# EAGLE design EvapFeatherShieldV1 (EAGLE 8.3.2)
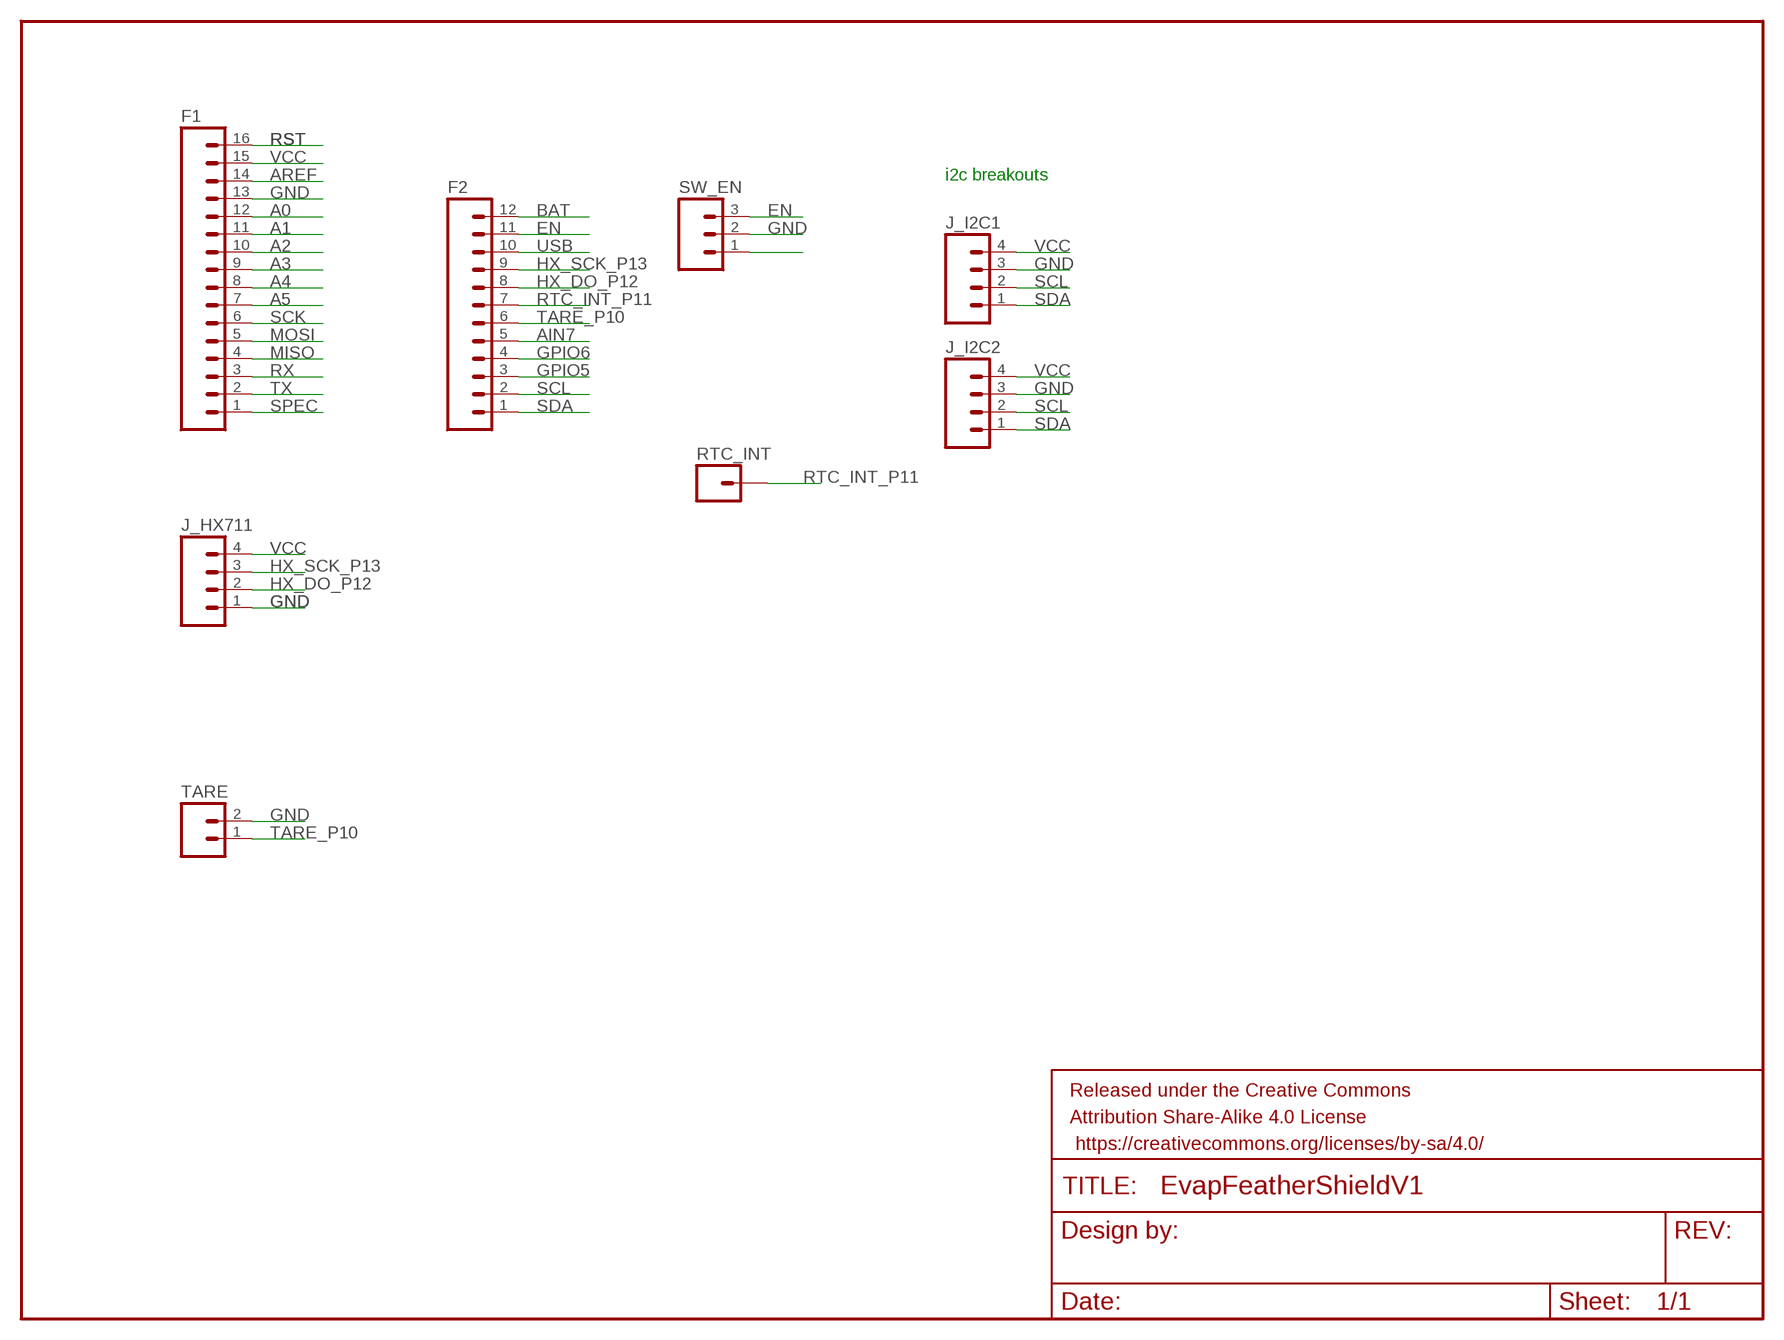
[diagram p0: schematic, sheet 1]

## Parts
F1  M16PTH  [1X16]
F2  M12PTH  [1X12]
FRAME1  FRAME-LETTER  [CREATIVE_COMMONS]
J_HX711  M04PTH  [1X04]
J_I2C1  M04PTH  [1X04]
J_I2C2  M04PTH  [1X04]
RTC_INT  M01PTH  [1X01]
SW_EN  M03PTH  [1X03]
TARE  M02PTH  [1X02]

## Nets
A0: F1.12
A1: F1.11
A2: F1.10
A3: F1.9
A4: F1.8
A5: F1.7
AIN7: F2.5
AREF: F1.14
BAT: F2.12
EN: F2.11 SW_EN.3
GND: F1.13 J_HX711.1 J_I2C1.3 J_I2C2.3 SW_EN.2 TARE.2
GPIO5: F2.3
GPIO6: F2.4
HX_DO_P12: F2.8 J_HX711.2
HX_SCK_P13: F2.9 J_HX711.3
MISO: F1.4
MOSI: F1.5
N$3: SW_EN.1
RST: F1.16
RTC_INT_P11: F2.7 RTC_INT.1
RX: F1.3
SCK: F1.6
SCL: F2.2 J_I2C1.2 J_I2C2.2
SDA: F2.1 J_I2C1.1 J_I2C2.1
SPEC: F1.1
TARE_P10: F2.6 TARE.1
TX: F1.2
USB: F2.10
VCC: F1.15 J_HX711.4 J_I2C1.4 J_I2C2.4

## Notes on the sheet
- i2c breakouts

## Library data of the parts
F1 = SparkFun-Connectors:M16: 1x16 .1" header
F2 = SparkFun-Connectors:M12: Header 12 Standard 12-pin 0.1" header. Use with straight break away headers (SKU : PRT-00116), right angle break away headers (PRT-00553), swiss pins (PRT-00743), machine pins (PRT-00117), and female headers (PRT-00115).
FRAME1 = SparkFun-Aesthetics:FRAME-LETTER: Schematic Frame
J_HX711 J_I2C1 J_I2C2 = SparkFun-Connectors:M04: Header 4 Standard 4-pin 0.1" header. Use with straight break away headers (SKU : PRT-00116), right angle break away headers (PRT-00553), swiss pins (PRT-00743), machine pins (PRT-00117), and female headers (PRT-00115). Molex polarized connector foot print use with SKU : PRT-08231 with associated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; PROD_ID: CONN-09696
RTC_INT = SparkFun-Connectors:M01: Header 1
SW_EN = SparkFun-Connectors:M03: Header 3 Standard 3-pin 0.1" header. Use with straight break away headers (SKU : PRT-00116), right angle break away headers (PRT-00553), swiss pins (PRT-00743), machine pins (PRT-00117), and female headers (PRT-00115). Molex polarized connector foot print use with SKU : PRT-08232 with associated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
TARE = SparkFun-Connectors:M02: Standard 2-pin 0.1" header. Use with

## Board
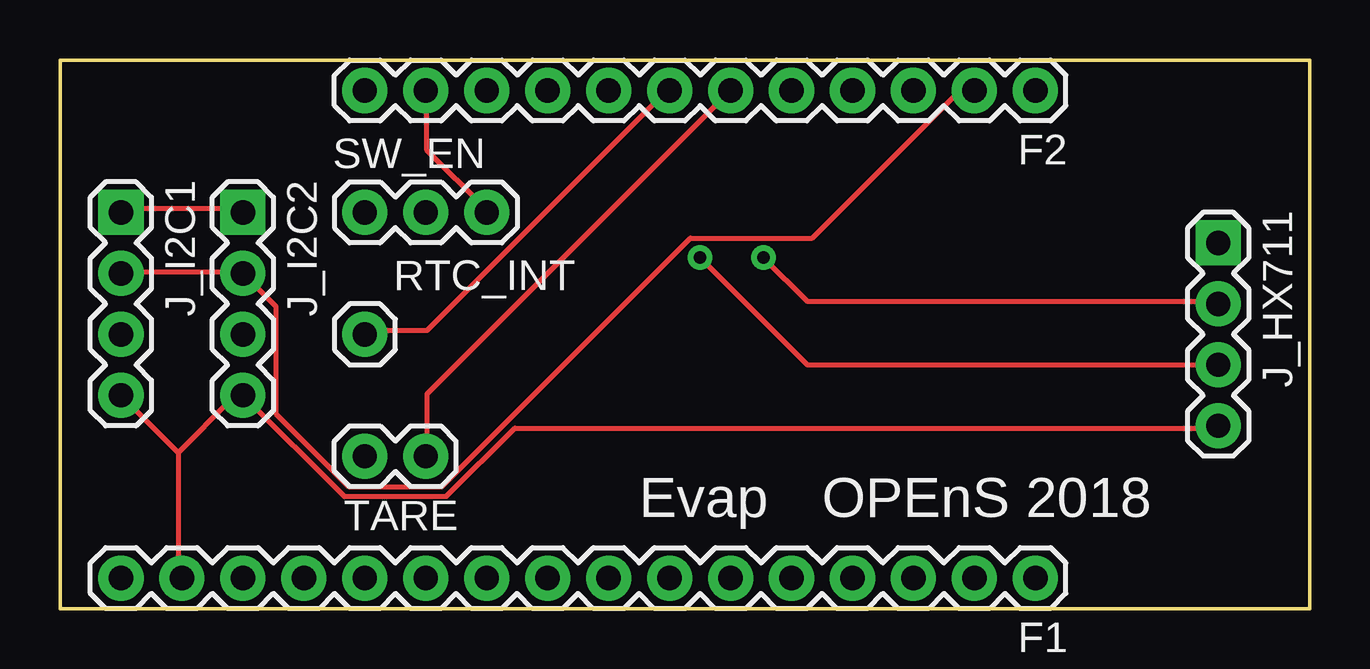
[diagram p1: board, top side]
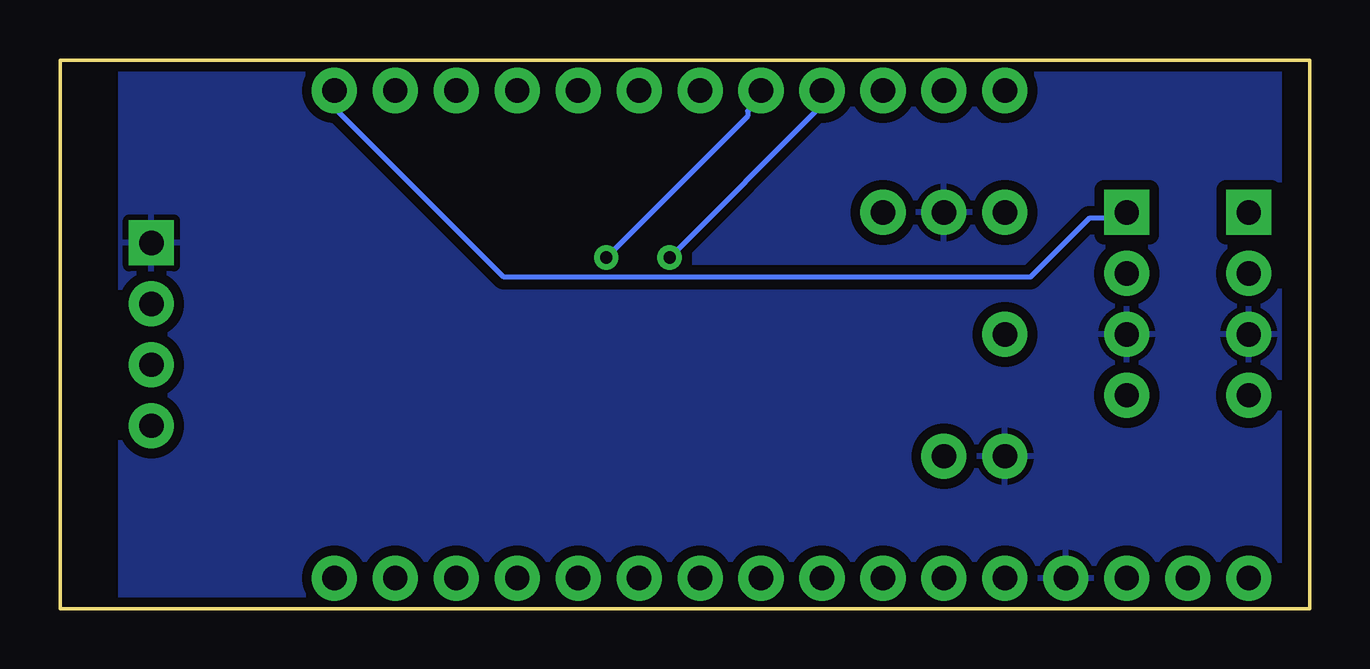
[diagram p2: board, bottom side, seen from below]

Size 52.07 x 22.86 mm. Coordinates in mm from the lower left corner, seen from the top.
Outline: 0,0 0,22.86 52.07,22.86 52.07,0 0,0
Copper layers (1*16): Top 0.035mm / dielectric 1.5mm / Bottom 0.035mm
Design rules "SparkFun": minimum track width 8mil, minimum drill 20mil, track to track 8mil, track to pad 8mil, pad to pad 8mil, via to via 8mil, smd to smd 8mil, copper to edge 8mil, drill to drill 8mil, minimum pad ring 12mil, minimum via ring 10mil, stop-mask expansion 4mil, vias tented up to drill 20mil, thermal gap 10mil

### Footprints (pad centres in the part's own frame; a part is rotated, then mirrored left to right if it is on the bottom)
1X16 = drill 1.016 pad 1.88: 1 0,0; 2 2.54,0; 3 5.08,0; 4 7.62,0; 5 10.16,0; 6 12.7,0; 7 15.24,0; 8 17.78,0; 9 20.32,0; 10 22.86,0; 11 25.4,0; 12 27.94,0; 13 30.48,0; 14 33.02,0; 15 35.56,0; 16 38.1,0
1X12 = drill 1.016 pad 1.88: 1 0,0; 2 2.54,0; 3 5.08,0; 4 7.62,0; 5 10.16,0; 6 12.7,0; 7 15.24,0; 8 17.78,0; 9 20.32,0; 10 22.86,0; 11 25.4,0; 12 27.94,0
1X04 = drill 1.016 pad 1.88 square: 1 0,0 | drill 1.016 pad 1.88: 2 2.54,0; 3 5.08,0; 4 7.62,0
1X01 = drill 1.016 pad 1.88: 1 0,0
1X03 = drill 1.016 pad 1.88: 1 0,0; 2 2.54,0; 3 5.08,0
1X02 = drill 1.016 pad 1.88: 1 0,0; 2 2.54,0

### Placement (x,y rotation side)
F1  40.64,1.27 180 top
F2  40.64,21.59 180 top
FRAME1  not placed on the board
J_HX711  48.26,15.24 270 top
J_I2C1  2.54,16.51 270 top
J_I2C2  7.62,16.51 270 top
RTC_INT  12.7,11.43 0 top
SW_EN  12.7,16.51 0 top
TARE  15.24,6.35 180 top

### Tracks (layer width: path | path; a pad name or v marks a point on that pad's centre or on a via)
EN
  Top 0.203: F2.11 15.29,21.54 15.29,19.1 17.73,16.66 SW_EN.3
GND
  pour Bottom (isolate 0.406): 1.27,0 1.27,22.86 49.53,22.86 49.53,0
HX_DO_P12  (via drill 0.51)
  Top 0.203: v29.31,14.63 31.14,12.8 48.21,12.8 J_HX711.2
  Bottom 0.203: v29.31,14.63 23.42,20.52 23.42,20.73 23.01,21.13 23.01,21.54 F2.8
HX_SCK_P13  (via drill 0.51)
  Top 0.203: J_HX711.3 31.14,10.16 v26.67,14.63
  Bottom 0.203: v26.67,14.63 20.37,20.93 20.37,21.54 F2.9
RTC_INT_P11
  Top 0.203: RTC_INT.1 12.85,11.58 15.29,11.58 25.25,21.54 F2.7
SCL
  Top 0.203: J_I2C1.2 2.69,14.02 7.57,14.02 J_I2C2.2 8.99,12.6 8.99,8.13 12.04,5.08 15.9,5.08 26.26,15.44 31.34,15.44 37.44,21.54 38.05,21.54 F2.2
SDA
  Top 0.203: J_I2C1.1 2.69,16.66 7.57,16.66 J_I2C2.1
  Bottom 0.203: F2.1 40.49,21.54 40.49,20.73 33.58,13.82 11.63,13.82 9.2,16.26 7.98,16.26 7.77,16.46 J_I2C2.1
TARE_P10
  Top 0.203: F2.6 15.29,8.94 15.29,6.5 TARE.1
VCC
  Top 0.203: 4.93,6.5 4.93,1.42 F1.15 | J_I2C1.4 4.93,6.5 | 4.93,6.5 7.16,8.74 7.57,8.74 J_I2C2.4 11.84,4.67 16.1,4.67 18.95,7.52 48.21,7.52 J_HX711.4

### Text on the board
tPlace: Evap | OPEnS 2018

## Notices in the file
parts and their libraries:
SparkFun-Aesthetics: Licensing: Creative Commons ShareAlike 4.0 International - https://creativecommons.org/licenses/by-sa/4.0
SparkFun-Aesthetics: Released under the Creative Commons Attribution Share-Alike 4.0 License
SparkFun-Aesthetics: https://creativecommons.org/licenses/by-sa/4.0
